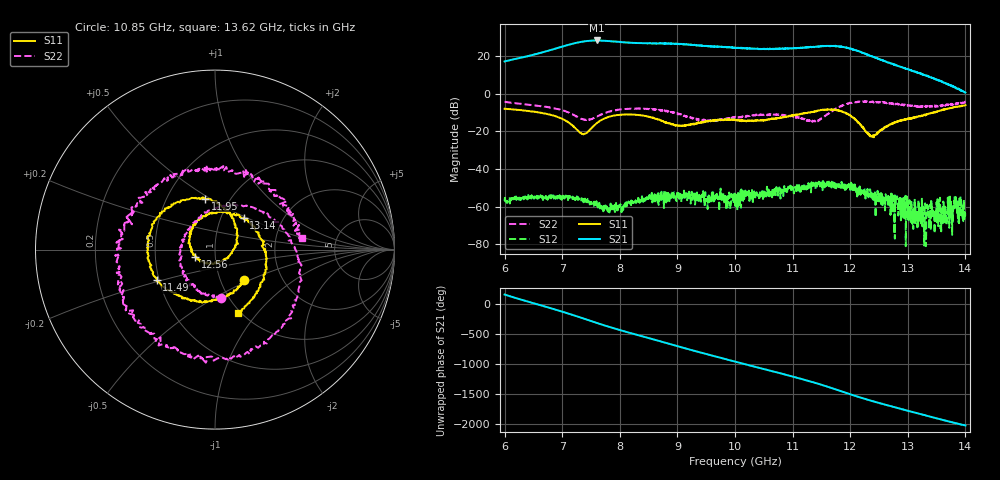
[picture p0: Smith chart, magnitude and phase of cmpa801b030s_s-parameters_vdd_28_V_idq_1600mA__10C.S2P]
!Keysight Technologies,E5071C,MY46110325,B.14.03
!Date: Fri Aug 07 13:41:26 2020
!Data & Calibration Information:
!Freq	S11:SOLT2(ON)	S21:SOLT2(ON)	S12:SOLT2(ON)	S22:SOLT2(ON)
!PortZ  Port1:50+j0  Port2:50+j0
!Above PortZ is port z conversion or system Z0 setting when saving the data.
!When reading, reference impedance value at option line is always used.
# Hz S dB R 50
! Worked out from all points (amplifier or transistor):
!   1601 points, 6 GHz to 14 GHz, reference 50 ohm
!   highest |S21| = 28.2 dB at 7.6 GHz (marker M1)
!   |S21| within 3 dB of that: 7.027 GHz to 9.518 GHz (2.491 GHz wide, 30.1 % of centre)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
!   unconditionally stable (mu >= 1): start of sweep to end of sweep
!   at 7.33 GHz: K = 13.69, MAG = 27.6 dB, |S12| = -56.6 dB
!   at 10 GHz: K = 20.93, MAG = 24.7 dB, |S12| = -57.5 dB
!   at 14 GHz: K = 276.78, MAG = 3.7 dB, |S12| = -61.6 dB
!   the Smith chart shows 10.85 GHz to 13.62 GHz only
!   S11 on the Smith chart (normalised r, x): 10.85 GHz: 1.29, -0.47; 11.49 GHz: 0.49, -0.19; 11.95 GHz: 0.77, +0.48; 12.56 GHz: 0.80, -0.07; 13.14 GHz: 1.28, +0.48; 13.62 GHz: 0.97, -0.79
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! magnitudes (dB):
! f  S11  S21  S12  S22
! 6 GHz  -8.1  17.0  -56.9  -4.4
! 6.865 GHz  -11.8  23.6  -55.1  -7.9
! 7.335 GHz  -21.3  27.5  -55.5  -13.4
! 7.6 GHz  -15.7  28.2  -59.8  -12.1
! 8.065 GHz  -11.1  27.2  -58.6  -8.3
! 8.67 GHz  -13.9  26.6  -57.6  -8.6
! 9.05 GHz  -17.0  26.3  -53.7  -11.0
! 9.51 GHz  -14.8  25.2  -56.9  -14.0
! 10 GHz  -13.9  24.3  -57.5  -12.6
! 10.21 GHz  -14.6  24.0  -53.7  -12.1
! 10.85 GHz  -12.6  23.7  -50.8  -11.4
! 11.34 GHz  -9.9  24.7  -48.9  -14.7
! 11.49 GHz  -8.8  25.0  -48.1  -13.4
! 11.95 GHz  -10.8  24.3  -50.0  -5.6
! 12.35 GHz  -22.6  19.9  -51.3  -4.4
! 12.56 GHz  -18.7  17.6  -57.3  -4.6
! 12.67 GHz  -16.8  16.5  -54.9  -4.9
! 12.83 GHz  -14.6  14.6  -61.0  -5.6
! 13.14 GHz  -12.4  11.6  -62.8  -6.8
! 13.62 GHz  -8.6  5.9  -57.8  -6.2
! 13.82 GHz  -7.2  3.2  -56.5  -5.8
! 14 GHz  -6.1  0.6  -61.6  -4.5
